FUNCTION FC 90 : VOID
TITLE =ALLARMI
VERSION : 0.1

BEGIN
NETWORK
TITLE =EMERGENZA INSERITA
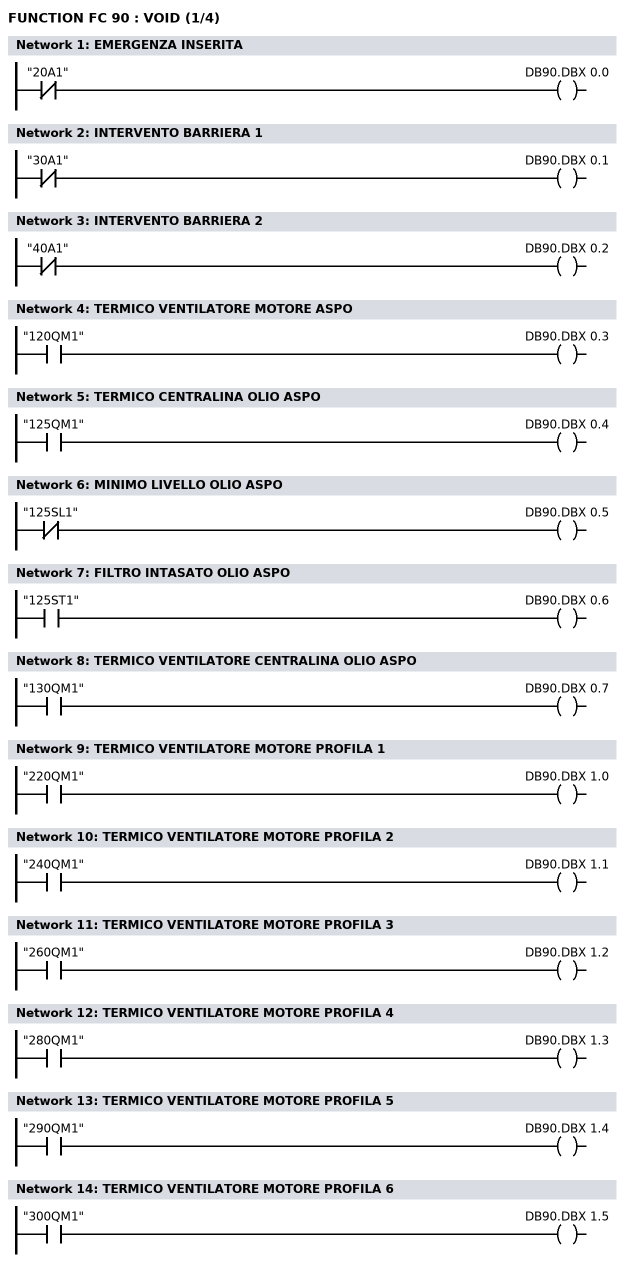
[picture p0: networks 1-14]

      UN    "20A1";
      =     DB90.DBX    0.0;
NETWORK
TITLE =INTERVENTO BARRIERA 1

      UN    "30A1";
      =     DB90.DBX    0.1;
NETWORK
TITLE =INTERVENTO BARRIERA 2

      UN    "40A1";
      =     DB90.DBX    0.2;
NETWORK
TITLE =TERMICO VENTILATORE MOTORE ASPO

      U     "120QM1";
      =     DB90.DBX    0.3;
NETWORK
TITLE =TERMICO CENTRALINA OLIO ASPO

      U     "125QM1";
      =     DB90.DBX    0.4;
NETWORK
TITLE =MINIMO LIVELLO OLIO ASPO

      UN    "125SL1";
      =     DB90.DBX    0.5;
NETWORK
TITLE =FILTRO INTASATO OLIO ASPO

      U     "125ST1";
      =     DB90.DBX    0.6;
NETWORK
TITLE =TERMICO VENTILATORE CENTRALINA OLIO ASPO

      U     "130QM1";
      =     DB90.DBX    0.7;
NETWORK
TITLE =TERMICO VENTILATORE MOTORE PROFILA 1

      U     "220QM1";
      =     DB90.DBX    1.0;
NETWORK
TITLE =TERMICO VENTILATORE MOTORE PROFILA 2

      U     "240QM1";
      =     DB90.DBX    1.1;
NETWORK
TITLE =TERMICO VENTILATORE MOTORE PROFILA 3

      U     "260QM1";
      =     DB90.DBX    1.2;
NETWORK
TITLE =TERMICO VENTILATORE MOTORE PROFILA 4

      U     "280QM1";
      =     DB90.DBX    1.3;
NETWORK
TITLE =TERMICO VENTILATORE MOTORE PROFILA 5

      U     "290QM1";
      =     DB90.DBX    1.4;
NETWORK
TITLE =TERMICO VENTILATORE MOTORE PROFILA 6

      U     "300QM1";
      =     DB90.DBX    1.5;
NETWORK
TITLE =TERMICO MOTORE CENTRALINA OLIO CESOIA
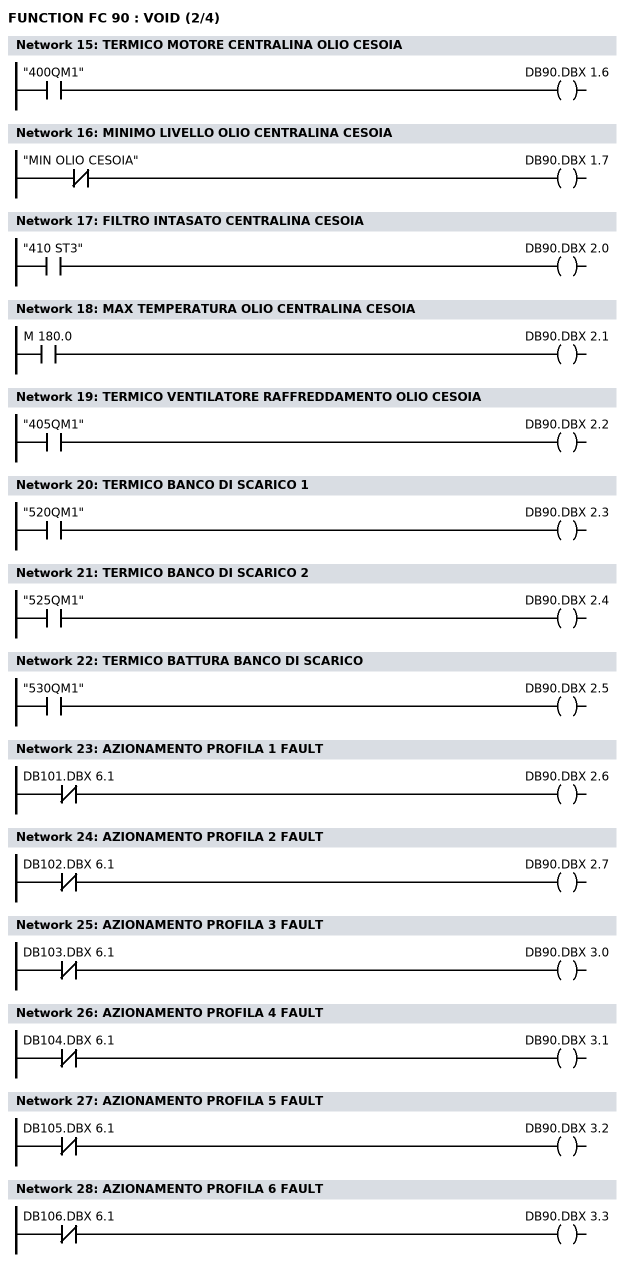
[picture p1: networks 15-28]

      U     "400QM1";
      =     DB90.DBX    1.6;
NETWORK
TITLE =MINIMO LIVELLO OLIO CENTRALINA CESOIA

      UN    "MIN OLIO CESOIA";
      =     DB90.DBX    1.7;
NETWORK
TITLE =FILTRO INTASATO CENTRALINA CESOIA

      U     "410 ST3";
      =     DB90.DBX    2.0;
NETWORK
TITLE =MAX TEMPERATURA OLIO CENTRALINA CESOIA

      U     M    180.0;
      =     DB90.DBX    2.1;
NETWORK
TITLE =TERMICO VENTILATORE RAFFREDDAMENTO OLIO CESOIA

      U     "405QM1";
      =     DB90.DBX    2.2;
NETWORK
TITLE =TERMICO BANCO DI SCARICO 1

      U     "520QM1";
      =     DB90.DBX    2.3;
NETWORK
TITLE =TERMICO BANCO DI SCARICO 2

      U     "525QM1";
      =     DB90.DBX    2.4;
NETWORK
TITLE =TERMICO BATTURA BANCO DI SCARICO

      U     "530QM1";
      =     DB90.DBX    2.5;
NETWORK
TITLE =AZIONAMENTO PROFILA 1 FAULT

      UN    DB101.DBX    6.1;
      =     DB90.DBX    2.6;
NETWORK
TITLE =AZIONAMENTO PROFILA 2 FAULT

      UN    DB102.DBX    6.1;
      =     DB90.DBX    2.7;
NETWORK
TITLE =AZIONAMENTO PROFILA 3 FAULT

      UN    DB103.DBX    6.1;
      =     DB90.DBX    3.0;
NETWORK
TITLE =AZIONAMENTO PROFILA 4 FAULT

      UN    DB104.DBX    6.1;
      =     DB90.DBX    3.1;
NETWORK
TITLE =AZIONAMENTO PROFILA 5 FAULT

      UN    DB105.DBX    6.1;
      =     DB90.DBX    3.2;
NETWORK
TITLE =AZIONAMENTO PROFILA 6 FAULT

      UN    DB106.DBX    6.1;
      =     DB90.DBX    3.3;
NETWORK
TITLE =AZIONAMENTO ASPO FAULT
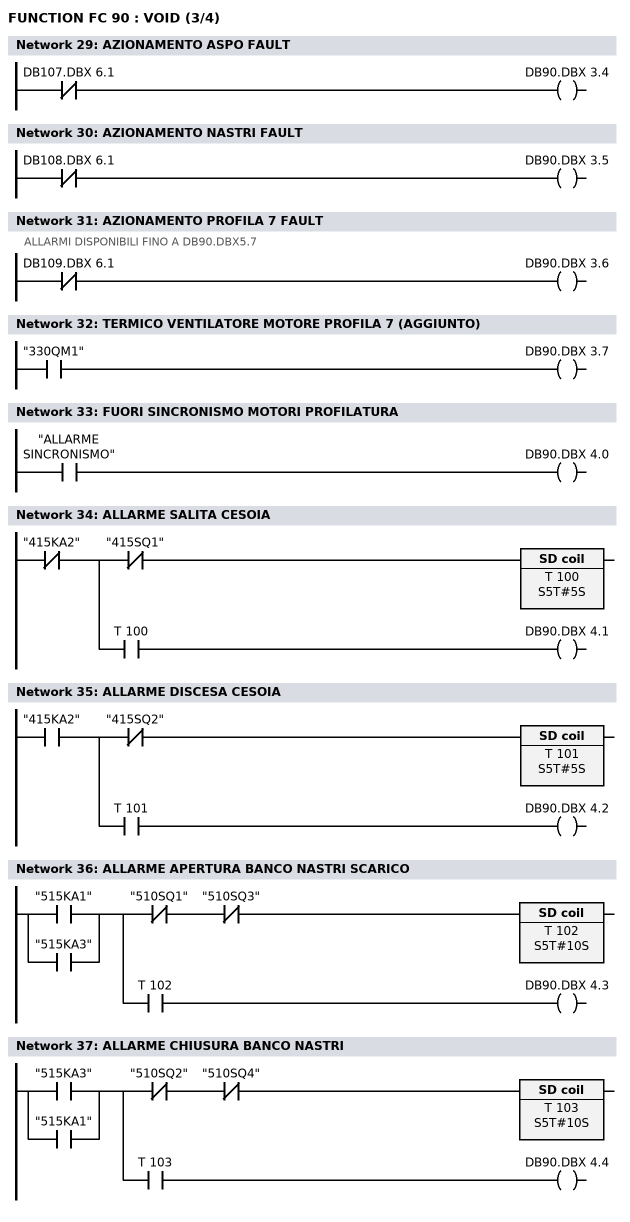
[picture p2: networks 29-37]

      UN    DB107.DBX    6.1;
      =     DB90.DBX    3.4;
NETWORK
TITLE =AZIONAMENTO NASTRI FAULT

      UN    DB108.DBX    6.1;
      =     DB90.DBX    3.5;
NETWORK
TITLE =AZIONAMENTO PROFILA 7 FAULT
//ALLARMI DISPONIBILI FINO A DB90.DBX5.7
      UN    DB109.DBX    6.1;
      =     DB90.DBX    3.6;
NETWORK
TITLE =TERMICO VENTILATORE MOTORE PROFILA 7 (AGGIUNTO)

      U     "330QM1";
      =     DB90.DBX    3.7;
NETWORK
TITLE =FUORI SINCRONISMO MOTORI PROFILATURA

      U     "ALLARME SINCRONISMO";
      =     DB90.DBX    4.0;
NETWORK
TITLE =ALLARME SALITA CESOIA

      UN    "415KA2";
      =     L      0.0;
      U     L      0.0;
      UN    "415SQ1";
      L     S5T#5S;
      SE    T    100;
      U     L      0.0;
      U     T    100;
      =     DB90.DBX    4.1;
NETWORK
TITLE =ALLARME DISCESA CESOIA

      U     "415KA2";
      =     L      0.0;
      U     L      0.0;
      UN    "415SQ2";
      L     S5T#5S;
      SE    T    101;
      U     L      0.0;
      U     T    101;
      =     DB90.DBX    4.2;
NETWORK
TITLE =ALLARME APERTURA BANCO NASTRI SCARICO

      O     "515KA1";
      O     "515KA3";
      =     L      0.0;
      U     L      0.0;
      UN    "510SQ1";
      UN    "510SQ3";
      L     S5T#10S;
      SE    T    102;
      U     L      0.0;
      U     T    102;
      =     DB90.DBX    4.3;
NETWORK
TITLE =ALLARME CHIUSURA BANCO NASTRI

      O     "515KA3";
      O     "515KA1";
      =     L      0.0;
      U     L      0.0;
      UN    "510SQ2";
      UN    "510SQ4";
      L     S5T#10S;
      SE    T    103;
      U     L      0.0;
      U     T    103;
      =     DB90.DBX    4.4;
NETWORK
TITLE =AZIONAMENTO PROFILA 8 FAULT
//ALLARMI DISPONIBILI FINO A DB90.DBX5.7
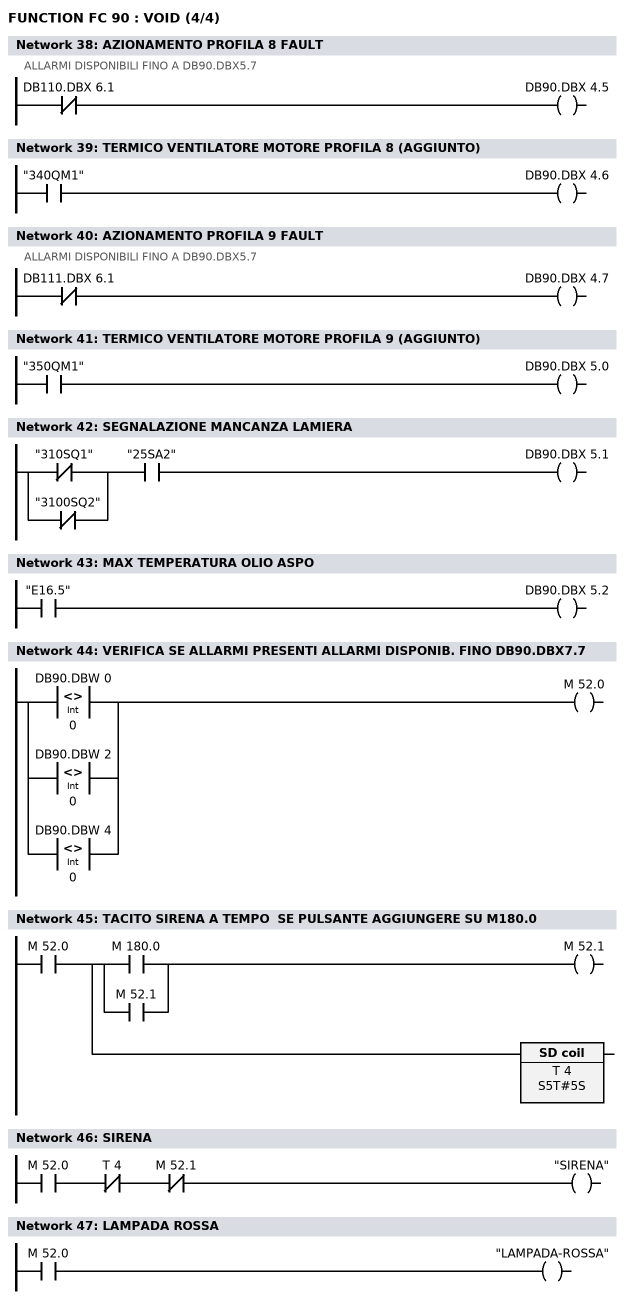
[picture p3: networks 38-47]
      UN    DB110.DBX    6.1;
      =     DB90.DBX    4.5;
NETWORK
TITLE =TERMICO VENTILATORE MOTORE PROFILA 8 (AGGIUNTO)

      U     "340QM1";
      =     DB90.DBX    4.6;
NETWORK
TITLE =AZIONAMENTO PROFILA 9 FAULT
//ALLARMI DISPONIBILI FINO A DB90.DBX5.7
      UN    DB111.DBX    6.1;
      =     DB90.DBX    4.7;
NETWORK
TITLE =TERMICO VENTILATORE MOTORE PROFILA 9 (AGGIUNTO)

      U     "350QM1";
      =     DB90.DBX    5.0;
NETWORK
TITLE =SEGNALAZIONE MANCANZA LAMIERA

      UN    "310SQ1";
      ON    "3100SQ2";
      U     "25SA2";
      =     DB90.DBX    5.1;
NETWORK
TITLE =MAX TEMPERATURA OLIO ASPO

      U     "E16.5";
      =     DB90.DBX    5.2;
NETWORK
TITLE =VERIFICA SE ALLARMI PRESENTI ALLARMI DISPONIB. FINO DB90.DBX7.7

      O(    ;
      L     DB90.DBW    0;
      L     0;
      <>I   ;
      )     ;
      O(    ;
      L     DB90.DBW    2;
      L     0;
      <>I   ;
      )     ;
      O(    ;
      L     DB90.DBW    4;
      L     0;
      <>I   ;
      )     ;
      =     M     52.0;
NETWORK
TITLE =TACITO SIRENA A TEMPO  SE PULSANTE AGGIUNGERE SU M180.0

      U     M     52.0;
      =     L      0.0;
      U     L      0.0;
      U(    ;
      O     M    180.0;
      O     M     52.1;
      )     ;
      =     M     52.1;
      U     L      0.0;
      BLD   102;
      L     S5T#5S;
      SE    T      4;
NETWORK
TITLE =SIRENA

      U     M     52.0;
      UN    T      4;
      UN    M     52.1;
      =     "SIRENA";
NETWORK
TITLE =LAMPADA ROSSA

      U     M     52.0;
      =     "LAMPADA-ROSSA";
END_FUNCTION

